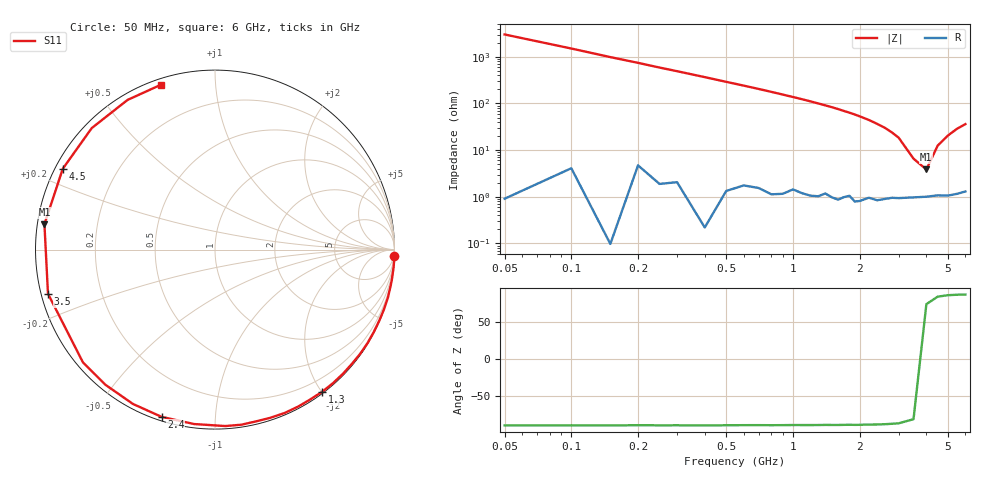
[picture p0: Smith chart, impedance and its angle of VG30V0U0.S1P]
! Infineon Technologies  Discrete & RF Semiconductors
! BB 831
! Si Tuning Diode in SOD323
! VR = 30 V
! S-Parameters:  July  1999
# GHz  S  MA  R  50
!  f  S11
! GHz  MAG  ANG
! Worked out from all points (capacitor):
!   34 points, 50 MHz to 6 GHz, reference 50 ohm
!   read as one part to ground: C = 1.06 pF near 50 MHz
!   lowest |Z| = 3.85 ohm at 4 GHz (marker M1)
!   series resonance near 3.818 GHz, so ESL is about 1.6 nH
!   S11 on the Smith chart (normalised r, x): 50 MHz: 0, -60; 1.3 GHz: 0.02, -2.01; 2.4 GHz: 0.02, -0.73; 3.5 GHz: 0.02, -0.13; 4.5 GHz: 0.02, +0.25; 6 GHz: 0.03, +0.72
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0.05  1 -1.9
0.15  1 -5.8
0.25  0.9995 -9.7
0.4  0.9998 -15.5
0.5  0.9985 -19.5
0.6  0.9971 -23.4
0.7  0.9965 -27.4
0.8  0.9967 -31.5
0.9  0.9957 -35.7
1.1  0.9933 -44.1
1.2  0.9929 -48.5
1.3  0.9919 -53.0
1.5  0.9897 -62.0
1.6  0.9895 -66.8
1.7  0.9865 -71.8
1.9  0.9866 -81.4
2  0.9848 -86.6
2.2  0.9788 -96.8
2.4  0.9783 -107.7
2.6  0.9739 -118.0
2.8  0.9694 -129.0
3  0.9676 -139.5
3.5  0.9625 -165.2
4  0.9608 171.5
4.5  0.9603 152.0
5  0.9643 135.4
5.5  0.9658 120.3
6  0.9664 108.3
